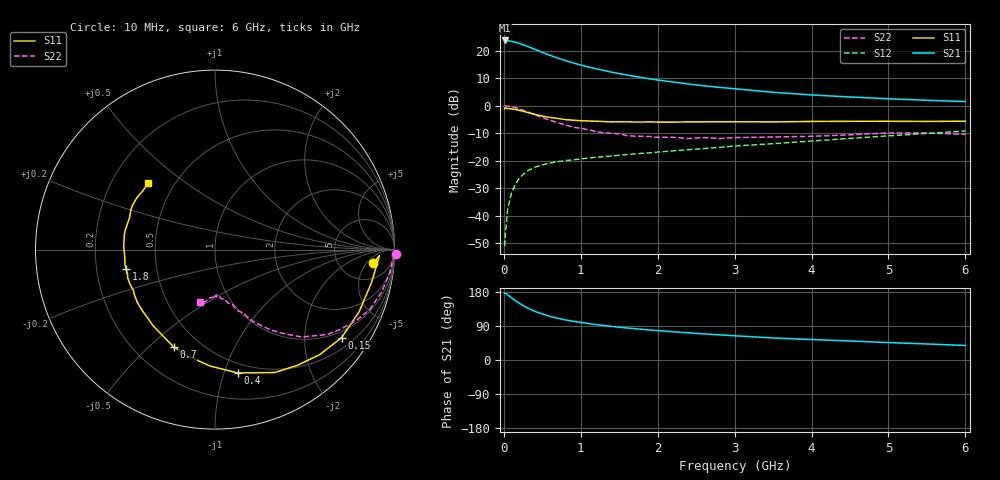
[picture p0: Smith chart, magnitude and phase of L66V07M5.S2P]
!  INFINEON TECHNOLOGIES Small Signal Semiconductors
! BFR380L3 , Si-NPN RF-Transistor in TSLP-3-1
!  Vce=6 V,  Ic=7.5 mA
! Common Emitter S-Parameters:  07. March 2005
#  GHz  S  MA  R  50
! f  S11  S21  S12  S22
! GHz  Mag  Ang  Mag  Ang  Mag  Ang  Mag  Ang
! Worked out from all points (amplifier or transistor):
!   36 points, 10 MHz to 6 GHz, reference 50 ohm
!   highest |S21| = 23.7 dB at 10 MHz (marker M1)
!   |S21| within 3 dB of that: start of sweep to 382.3 MHz
!   unconditionally stable (mu >= 1): 2.765 GHz to 2.949 GHz; 3.016 GHz to 4.56 GHz
!   at 250 MHz: K = 0.18, MSG = 23.6 dB, |S12| = -25.0 dB
!   at 1.4 GHz: K = 0.76, MSG = 15.3 dB, |S12| = -18.3 dB
!   at 6 GHz: K = 0.94, MSG = 5.4 dB, |S12| = -9.2 dB
!   S11 on the Smith chart (normalised r, x): 10 MHz: 11, -8; 150 MHz: 0.80, -3.00; 400 MHz: 0.41, -1.11; 700 MHz: 0.36, -0.60; 1.8 GHz: 0.33, -0.10; 6 GHz: 0.36, +0.37
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0.01  0.8851 -4.8  15.39 176.5  0.0028 75.8  1.008 -1.5
0.02  0.9171 -2.1  15.29 176.9  0.0046 86.2  0.9923 -3.0
0.05  0.8912 -11.9  15.22 172.0  0.0134 85.6  0.983 -7.3
0.1  0.8748 -23.2  14.8 164.4  0.026 78.2  0.958 -14.3
0.15  0.8591 -34.8  14.34 156.9  0.0377 72.4  0.9245 -21.2
0.2  0.8263 -45.1  13.63 149.9  0.0479 67.9  0.8804 -26.7
0.25  0.7919 -54.4  12.88 144.0  0.0563 63.1  0.8291 -32.3
0.3  0.7618 -64.0  12.09 138.2  0.0647 59.8  0.7841 -37.1
0.4  0.6991 -79.5  10.66 128.7  0.0761 53.9  0.6875 -45.1
0.5  0.6492 -92.4  9.362 121.4  0.0842 50.4  0.6096 -50.4
0.6  0.6124 -104.1  8.254 115.0  0.0911 47.5  0.5459 -55.2
0.7  0.5885 -113.1  7.373 110.2  0.0962 46.2  0.4924 -58.9
0.9  0.5466 -129.2  6.014 102.2  0.1042 44.8  0.4084 -64.8
1.1  0.5286 -140.3  5.073 96.0  0.1123 45.0  0.3668 -69.1
1.4  0.5082 -153.7  4.085 88.8  0.1217 45.9  0.3171 -73.6
1.8  0.5066 -167.6  3.252 80.8  0.1367 48.3  0.2789 -79.7
2.2  0.5048 -177.3  2.7 74.5  0.1514 50.7  0.2673 -84.1
2.8  0.512 170.4  2.162 66.4  0.1751 54.1  0.2528 -91.4
3.5  0.5081 159.7  1.758 58.1  0.2045 55.8  0.2706 -95.9
4.5  0.5218 151.0  1.444 50.2  0.2553 58.7  0.2965 -100.8
5.5  0.5186 141.1  1.258 42.3  0.3143 58.4  0.3207 -104.8
6  0.5245 135.0  1.192 38.4  0.3476 57.5  0.3021 -106.3
